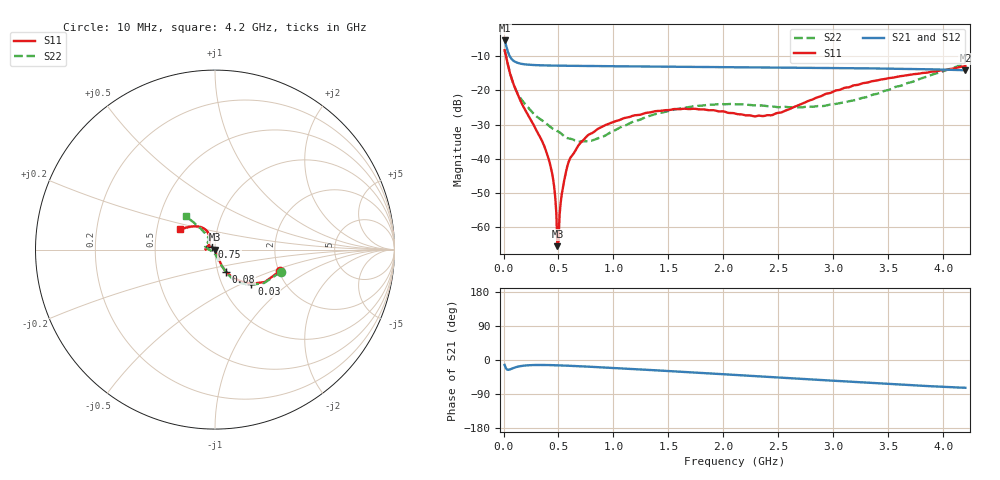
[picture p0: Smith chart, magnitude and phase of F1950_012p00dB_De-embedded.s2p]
! Integrated Device Technology
! Corporate Headquarters
! 6024 Silver Creek Valley Road
! San Jose, CA 95138  USA
! Phone:  1-408-284-8200
! Toll Free:  1-800-223-1366
! Webpage:  http://www.idt.com/
! Timing and RF Division
! 515 Groton Road, Suite 102
! Westford, MA 01886-6024
! Device:  F1950
! Description: 7-bit 0.25 dB Digital Step Attenuator
! Frequency:  150.0 -  4000.00 MHz
! Package:  4x4 mm Thin QFN Plastic Package: 24 pin
! Ports:  2 RF, 12 DC
!  Pin  1  = D0
!  Pin  2  = VDD
!  Pin  3  = Vmode
!  Pin  4  = GND
!  Pin  5  = RF1  =  Port 1
!  Pin  6  = GND
!  Pin  7  = GND
!  Pin  8  = GND
!  Pin  9  = GND
!  Pin 10  = GND
!  Pin 11  = GND
!  Pin 12  = GND
!  Pin 13  = GND
!  Pin 14  = RF2  =  Port 2
!  Pin 15  = GND
!  Pin 16  = LE
!  Pin 17  = CLK
!  Pin 18  = DATE
!  Pin 19  = D6
!  Pin 20  = D5
!  Pin 21  = D4
!  Pin 22  = D3
!  Pin 23  = D2
!  Pin 24  = D1
! State:  48
! Atten State:  12.00 dB
! Voltage:  +5.00 Volts
! Current:  Not Measured mA
! Data:  The device was measured on a the F195X evaluation board which has
!  individual transmission lines to the RF pins.  Data was collected
!  using a calibrated network analyzer.  The evaluation board was
!  de-embedded using a TRL calibration technique.
!  The reference plane is the edge of the package pin.
! Misc:  Board 2019
!  Action Tracker AT0250
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# GHz S dB R 50
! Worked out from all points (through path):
!   420 points, 10 MHz to 4.2 GHz, reference 50 ohm
!   highest |S21| = -5.49 dB at 10 MHz (marker M1); lowest = -14.2 dB at 4.2 GHz (marker M2)
!   group delay of S21, straight-line fit = 43.2 ps
!   lowest |S11| = -65.5 dB at 490 MHz (marker M3), VSWR 1.00, Z = 50 - j0.0518 ohm
!   |S11| at or under -10 dB: 22.63 MHz to end of sweep
!   |S22| runs from -35.0 to -8.3 dB; largest |S21 - S12| = 0.00032
!   S11 on the Smith chart (normalised r, x): 10 MHz: 2.04, -0.56; 30 MHz: 1.37, -0.57; 80 MHz: 1.10, -0.27; 750 MHz: 0.97, +0.03; 4.2 GHz: 0.66, +0.16
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0.01  -8.33 -17.9  -5.49 -12.8  -5.49 -12.8  -8.27 -18.9
0.03  -11.12 -43.2  -7.79 -24.7  -7.79 -24.7  -11.06 -44.6
0.08  -17.27 -63.3  -11.10 -22.3  -11.10 -22.3  -17.16 -64.1
0.18  -24.76 -66.8  -12.40 -15.1  -12.40 -15.1  -23.41 -72.1
0.34  -34.12 -61.8  -12.74 -13.1  -12.74 -13.1  -28.55 -78.3
0.4  -38.98 -59.5  -12.79 -13.3  -12.79 -13.3  -30.01 -79.7
0.45  -45.72 -58.6  -12.82 -13.7  -12.82 -13.7  -31.29 -84.5
0.48  -55.65 -60.2  -12.84 -13.9  -12.84 -13.9  -31.79 -88.3
0.49  -65.47 -76.4  -12.84 -14.0  -12.84 -14.0  -31.93 -89.3
0.51  -56.34 148.3  -12.85 -14.2  -12.85 -14.2  -32.28 -90.4
0.54  -48.40 140.1  -12.86 -14.5  -12.86 -14.5  -33.10 -92.7
0.59  -41.11 136.8  -12.88 -15.1  -12.88 -15.1  -34.03 -102.3
0.71  -35.04 141.2  -12.92 -16.7  -12.92 -16.7  -34.91 -122.8
0.75  -33.68 140.9  -12.93 -17.3  -12.93 -17.3  -34.87 -129.2
1.01  -29.12 154.7  -13.01 -21.2  -13.01 -21.2  -31.74 -169.6
1.41  -26.06 171.5  -13.12 -27.7  -13.11 -27.7  -26.70 169.5
1.73  -25.40 178.2  -13.19 -32.9  -13.19 -33.0  -24.68 160.7
2.11  -26.85 171.0  -13.28 -39.5  -13.28 -39.5  -24.11 151.4
2.44  -27.27 138.5  -13.36 -45.0  -13.35 -45.0  -24.71 141.3
2.81  -22.70 113.3  -13.45 -51.5  -13.45 -51.5  -24.84 126.4
3.51  -16.45 122.8  -13.70 -63.4  -13.70 -63.5  -19.84 120.7
4.2  -12.95 149.3  -14.18 -73.3  -14.18 -73.4  -12.13 131.1
